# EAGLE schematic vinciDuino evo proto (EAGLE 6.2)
Assembly variants: No 3.3V Reg
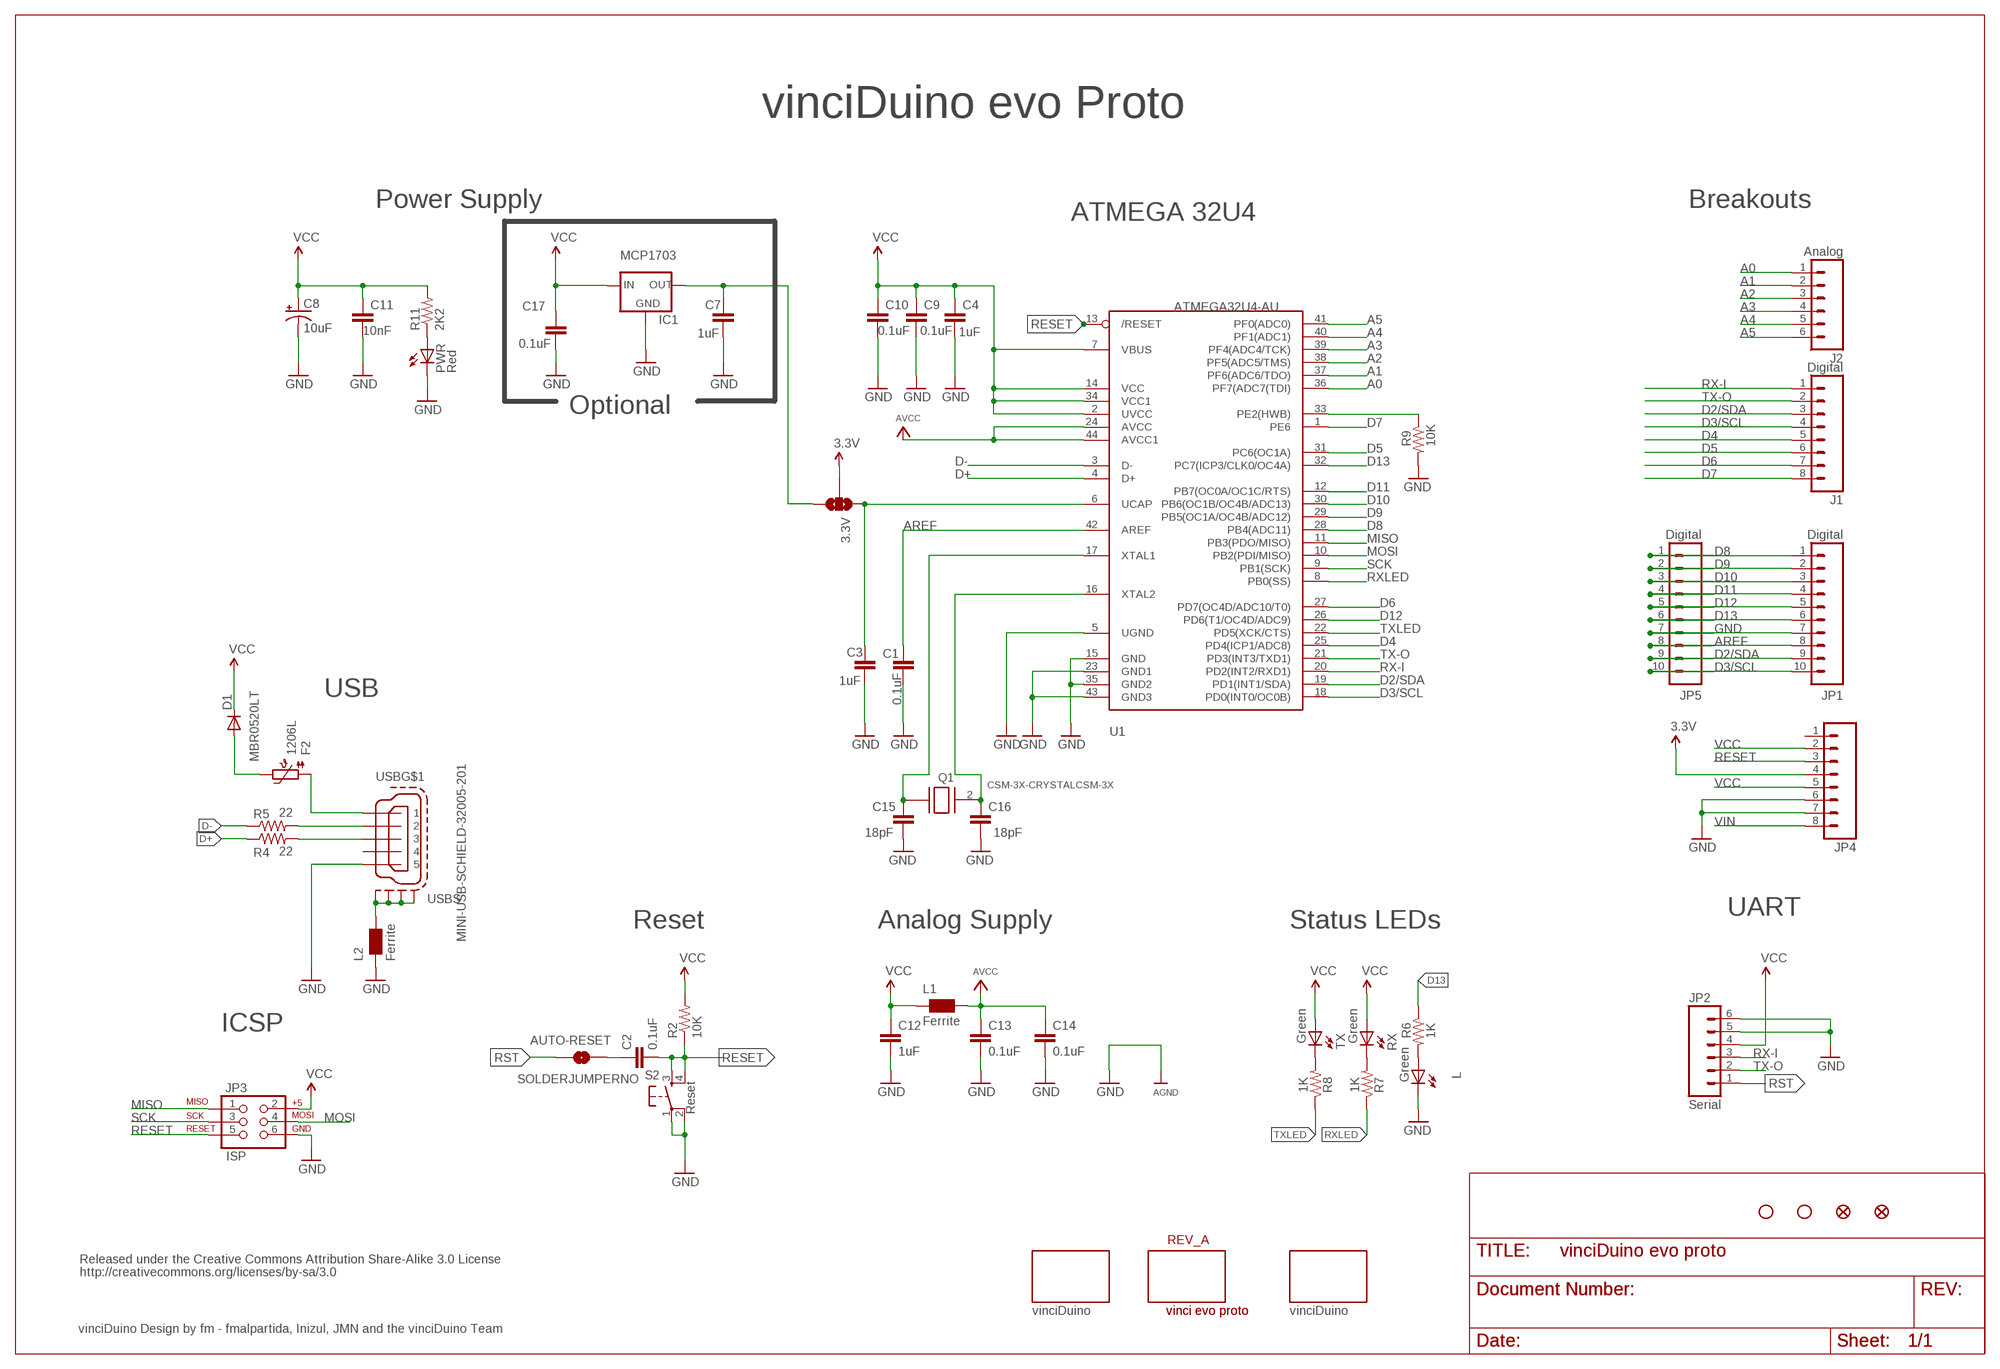
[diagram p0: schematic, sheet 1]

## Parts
3.3V  SOLDERJUMPER_2WAYS  [SJ_3]
AUTO-RESET  SOLDERJUMPERNO  [SJ_2S-NO]
C1  0.1uF  CAP1206  [1206]
C2  0.1uF  CAP1206  [1206]
C3  1uF  CAP1206  [1206]
C4  1uF  CAP1206  [1206]
C7  1uF  CAP1206  [1206]  (not fitted in variant No 3.3V Reg)
C8  10uF  CAP_POL1206  [EIA3216]
C9  0.1uF  CAP1206  [1206]
C10  0.1uF  CAP1206  [1206]
C11  10nF  CAP1206  [1206]
C12  1uF  CAP1206  [1206]
C13  0.1uF  CAP1206  [1206]
C14  0.1uF  CAP1206  [1206]
C15  18pF  CAP1206  [1206]
C16  18pF  CAP1206  [1206]
C17  0.1uF  CAP1206  [1206]  (not fitted in variant No 3.3V Reg)
D1  MBR0520LT  [SOD123]
F2  1206L  PTC1206_L  [1206_PTC]
IC1  MCP1703  V_REG_MIC2920  [SOT223]  (not fitted in variant No 3.3V Reg)
J1  Digital  M081X08  [1X08]
J2  Analog  M06SIP  [1X06]
JP1  Digital  M10"  [1X10]
JP2  Serial  M06SIP  [1X06]
JP3  ISP  AVR_SPI_PRG_6PTH  [2X3]
JP4  M081X08  [1X08]
JP5  Digital  M10"  [1X10]
L  Green  LED1206  [LED-1206]
L1  Ferrite  WE-CBF_1206W  [1206W]
L2  Ferrite  WE-CBF_1206W  [1206W]
PWR  Red  LED1206  [LED-1206]
Q1  CSM-3X-CRYSTALCSM-3X  [CSM-3X]
R2  10K  R-US_R1206  [R1206]
R4  22  R-US_R1206  [R1206]
R5  22  R-US_R1206  [R1206]
R6  1K  R-US_R1206  [R1206]
R7  1K  R-US_R1206  [R1206]
R8  1K  R-US_R1206  [R1206]
R9  10K  R-US_R1206  [R1206]
R11  2K2  R-US_R1206  [R1206]
REV_A  vinci evo proto  BOARD_INFO_  [ARDUINO_FORUM]
RX  Green  LED1206  [LED-1206]
S2  Reset  TAC_SWITCHSMD  [TACTILE_SWITCH_SMD]
TX  Green  LED1206  [LED-1206]
U1  ATMEGA32U4-AU  [TQFP44]
U$1  VINCIDUINO_  VINCIDUINO_25  [VINCIDUINO]
U$2  FIDUCIAL1X2  [FIDUCIAL-1X2]
U$3  VINCIDUINO_15  [VINCIDUINO_VSMAL]
U$4  FIDUCIAL1X2  [FIDUCIAL-1X2]
U$9  STAND-OFF  [STAND-OFF]
U$15  STAND-OFF  [STAND-OFF]
USB  MINI-USB-SCHIELD-32005-201  [32005-201]

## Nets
3.3V: 3.3V.2 JP4.4
A0: J2.1 U1.36(PF7(ADC7(TDI))
A1: J2.2 U1.37(PF6(ADC6/TDO))
A2: J2.3 U1.38(PF5(ADC5/TMS))
A3: J2.4 U1.39(PF4(ADC4/TCK))
A4: J2.5 U1.40(PF1(ADC1))
A5: J2.6 U1.41(PF0(ADC0))
AREF: C1.2 JP1.8 JP5.8 U1.42(AREF)
AVCC: C13.1 C14.1 L1.2 U1.24(AVCC) U1.44(AVCC1)
D2/SDA: J1.3 JP1.9 JP5.9 U1.19(PD1(INT1/SDA))
D3/SCL: J1.4 JP1.10 JP5.10 U1.18(PD0(INT0/OC0B))
D4: J1.5 U1.25(PD4(ICP1/ADC8))
D5: J1.6 U1.31(PC6(OC1A))
D6: J1.7 U1.27(PD7(OC4D/ADC10/T0))
D7: J1.8 U1.1(PE6)
D8: JP1.1 JP5.1 U1.28(PB4(ADC11))
D9: JP1.2 JP5.2 U1.29(PB5(OC1A/OC4B/ADC12))
D10: JP1.3 JP5.3 U1.30(PB6(OC1B/OC4B/ADC13))
D11: JP1.4 JP5.4 U1.12(PB7(OC0A/OC1C/RTS))
D12: JP1.5 JP5.5 U1.26(PD6(T1/OC4D/ADC9))
D13: JP1.6 JP5.6 R6.1 U1.32(PC7(ICP3/CLK0/OC4A))
D+: R4.1 U1.4(D+)
D-: R5.1 U1.3(D-)
GND: C1.1 C3.2 C4.2 C7.2 C8.C(-) C9.2 C10.2 C11.2 C12.2 C13.2 C14.2 C15.2 C16.2 C17.1 IC1.2(GND) JP1.7 JP2.5 JP2.6 JP3.6 JP4.6 JP4.7 JP5.7 L2.1 L.C PWR.C R9.2 S2.1 S2.2 U1.5(UGND) U1.15(GND) U1.23(GND1) U1.35(GND2) U1.43(GND3) USB.5 ; supply symbol labelled AGND
MISO: JP3.1 U1.11(PB3(PDO/MISO))
MOSI: JP3.4 U1.10(PB2(PDI/MISO))
N$1: R8.2 TX.C
N$2: R5.2 USB.2
N$3: C16.1 Q1.2 U1.16(XTAL2)
N$4: C15.1 Q1.1 U1.17(XTAL1)
N$5: R4.2 USB.3
N$6: R9.1 U1.33(PE2(HWB))
N$7: L.A R6.2
N$8: AUTO-RESET.2 C2.1
N$9: R7.2 RX.C
N$10: L2.2 USB.M1(S:S1) USB.M2(S:S2) USB.M3(S:S3) USB.M4(S:S4)
N$13: F2.1 USB.1
N$36: D1.A F2.2
N$38: PWR.A R11.1
N$94: 3.3V.1 C3.1 U1.6(UCAP)
N$840: 3.3V.3 C7.1 IC1.3(OUT)
RESET: C2.2 JP3.5 JP4.3 R2.1 S2.3 S2.4 U1.13(/RESET)
RST: AUTO-RESET.1 JP2.1
RX-I: J1.1 JP2.3 U1.20(PD2(INT2/RXD1))
RXLED: R7.1 U1.8(PB0(SS))
SCK: JP3.3 U1.9(PB1(SCK))
TX-O: J1.2 JP2.2 U1.21(PD3(INT3/TXD1))
TXLED: R8.1 U1.22(PD5(XCK/CTS))
VCC: C4.1 C8.A(+) C9.1 C10.1 C11.1 C12.1 C17.2 D1.C IC1.1(IN) JP2.4 JP3.2 JP4.2 JP4.5 L1.1 R2.2 R11.2 RX.A TX.A U1.2(UVCC) U1.7(VBUS) U1.14(VCC) U1.34(VCC1)
VIN [vcc]: JP4.8
Unconnected: JP4.1 USB.4

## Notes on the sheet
- vinciDuino evo Proto
- Power Supply | Breakouts
- ATMEGA 32U4
- Optional
- USB
- UART
- Reset | Analog Supply | Status LEDs
- ICSP
- Released under the Creative Commons Attribution Share-Alike 3.0 License
- http://creativecommons.org/licenses/by-sa/3.0
- vinciDuino Design by fm - fmalpartida, Inizul, JMN and the vinciDuino Team

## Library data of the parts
3.3V = SparkFun:SOLDERJUMPER_2WAY: Solder Jumper 2 way solder jumper
AUTO-RESET = SparkFun:SOLDERJUMPER: Solder Jumper
C1-C4 C7 C9-C17 = sparkfun_2:CAP: Capacitor
C8 = SparkFun:CAP_POL: Capacitor Polarized
D1 = diode:MBR0520LT: SCHOTTKY BARRIER RECTIFIER
F2 = microbuilder:PTC: PTC (Resettable Fuse)
IC1 = SparkFun:V_REG_MIC2920: MIC2920A (http://www.micrel.com/_PDF/mic2920.pdf) - 400mA output LDO Regulator
J1 JP4 = SparkFun:M08: Header 8 Standard 8-pin 0.1" header. Use with straight break away headers (SKU : PRT-00116), right angle break away headers (PRT-00553), swiss pins (PRT-00743), machine pins (PRT-00117), and female headers (PRT-00115).
J2 JP2 = SparkFun:M06: Header 6 Standard 6-pin 0.1" header. Use with straight break away headers (SKU : PRT-00116), right angle break away headers (PRT-00553), swiss pins (PRT-00743), machine pins (PRT-00117), and female headers (PRT-00115). Molex polarized connector foot print use with SKU : PRT-08094 with associated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
JP1 JP5 = SparkFun:M10: Header 10 Standard 10-pin 0.1" header. Use with straight break away headers (SKU : PRT-00116), right angle break away headers (PRT-00553), swiss pins (PRT-00743), machine pins (PRT-00117), and female headers (PRT-00115).
JP3 = SparkFun:AVR_SPI_PRG_6: AVR ISP 6 Pin This is the reduced ISP connector for AVR programming. Common on Arduino. This footprint will take up less PCB space and can be used with a 10-pin to 6-pin adapter such as SKU: BOB-08508
L PWR RX TX = SparkFun:LED: LEDs
L1 L2 = wuerth-elektronik:WE-CBF: SMD EMI Suppression Ferrite Beads
Q1 = fmc:CSM-3X-CRYSTAL
R2 R4-R9 R11 = adafruit:R-US_: RESISTOR, American symbol
REV_A = fmc:BOARD_INFO_
S2 = SparkFun:TAC_SWITCH: Momentary Switch Button commonly used for reset or general input. Spark Fun Electronics SKU : COM-00097
U1 = adafruit:ATMEGA32U4: http://www.ladyada.net/library/eagle
U$1 U$3 = fmc:VINCIDUINO_
U$2 U$4 = SparkFun:FIDUCIAL: Fiducial Alignment Points
U$9 U$15 = SparkFun:STAND-OFF: Stand Off
USB = con-cypressindustries:MINI-USB-SCHIELD-: MINI USB-B Conector Source: www.cypressindustries.com; OC_FARNELL: unknown; OC_NEWARK: unknown

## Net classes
1 vcc: width 0.254 mm
2 usb: width 0.203 mm, clearance 0.508 mm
